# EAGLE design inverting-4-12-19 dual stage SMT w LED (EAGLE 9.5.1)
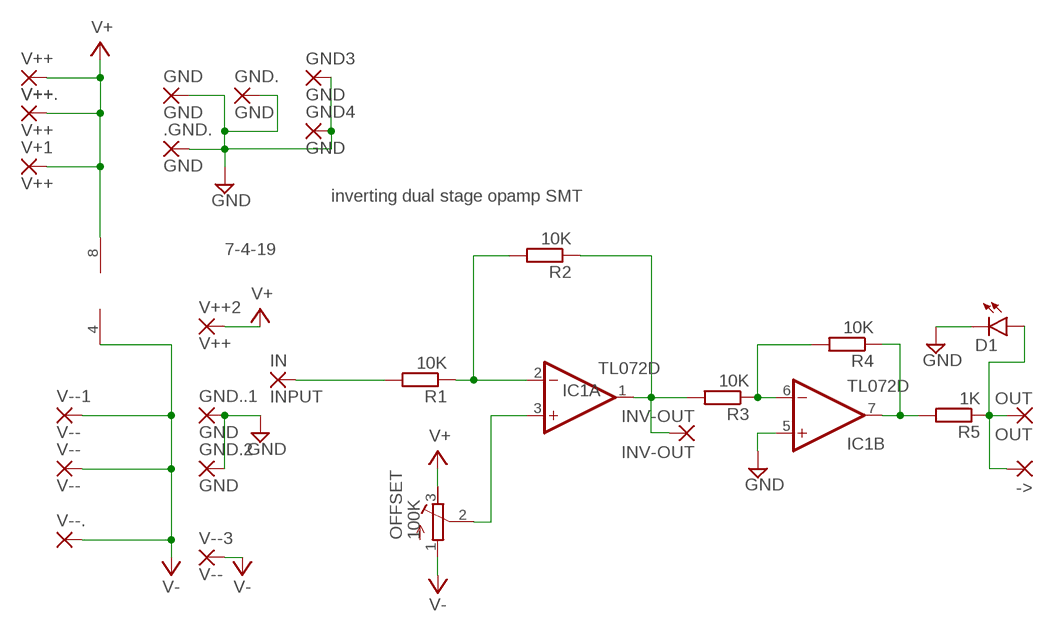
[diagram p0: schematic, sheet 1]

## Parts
->  1,6/0,8  [1,6/0,8]
.GND.  GND  1,6/0,9  [1,6/0,9]
D1  LED3MM  [LED3MM]
GND  GND  1,6/0,8  [1,6/0,8]
GND3  GND  1,6/0,8  [1,6/0,8]
GND4  GND  1,6/0,8  [1,6/0,8]
GND.  GND  1,6/0,8  [1,6/0,8]
GND.2  GND  1,6/0,8  [1,6/0,8]
GND..1  GND  1,6/0,8  [1,6/0,8]
IC1  TL072D  [SO08]
IN  INPUT  1,6/0,8  [1,6/0,8]
INV-OUT  INV-OUT  1,6/0,8  [1,6/0,8]
OFFSET  100K  R-TRIMM64W  [RTRIM64W]
OUT  OUT  1,6/0,8  [1,6/0,8]
R1  10K  RESISTORVERTICAL  [VERTICAL_RESISTOR]
R2  10K  RESISTORVERTICAL  [VERTICAL_RESISTOR]
R3  10K  RESISTORVERTICAL  [VERTICAL_RESISTOR]
R4  10K  RESISTORVERTICAL  [VERTICAL_RESISTOR]
R5  1K  RESISTORVERTICAL  [VERTICAL_RESISTOR]
V+1  V++  1,6/0,8  [1,6/0,8]
V++  V++  1,6/0,8  [1,6/0,8]
V++2  V++  1,6/0,8  [1,6/0,8]
V++.  V++  1,6/0,8  [1,6/0,8]
V--  V--  1,6/0,8  [1,6/0,8]
V--1  V--  1,6/0,8  [1,6/0,8]
V--3  V--  1,6/0,8  [1,6/0,8]
V--.  1,6/0,8  [1,6/0,8]

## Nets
GND: .GND..1(P) D1.K(C) GND3.1(P) GND4.1(P) GND.1(P) GND.2.1(P) GND..1(P) GND..1.1(P) IC1.5(B:+IN)
N$1: IC1.3(A:+IN) OFFSET.2(S)
N$2: ->.1(P) D1.A OUT.1(P) R5.1
N$3: IN.1(P) R1.2
N$5: IC1.2(A:-IN) R1.1 R2.2
N$6: IC1.6(B:-IN) R3.1 R4.2
N$7: IC1.7(B:OUT) R4.1 R5.2
N$18: IC1.1(A:OUT) INV-OUT.1(P) R2.1 R3.2
V+: IC1.8(P:V+) OFFSET.3(E) V+1.1(P) V++2.1(P) V++.1(P) V++..1(P)
V-: IC1.4(P:V-) OFFSET.1(A) V--1.1(P) V--3.1(P) V--.1(P) V--..1(P)

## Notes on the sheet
- inverting dual stage opamp SMT
- 7-4-19

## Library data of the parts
-> GND GND. IN INV-OUT OUT V++ V++. V-- V--. = wirepad:1,6/0,8: THROUGH-HOLE PAD
.GND. = wirepad:1,6/0,9: THROUGH-HOLE PAD
D1 = diodes:LED
GND3 GND4 GND.2 GND..1 V+1 V++2 V--1 V--3 = wirepad-NONAMES:1,6/0,8: THROUGH-HOLE PAD
IC1 = linear:TL072: OP AMP
OFFSET = rcl:R-TRIMM: Trimm resistor; SPICEMODEL: X; SPICEPREFIXL: POT
R1-R5 = MusicThingModular:RESISTOR: Standard resistor, various versions

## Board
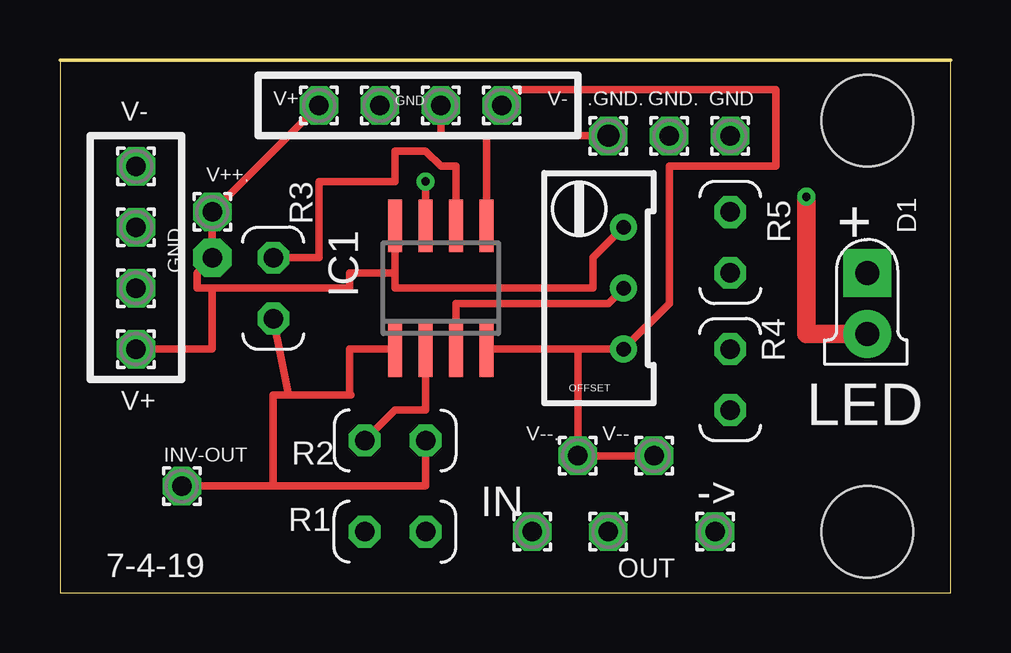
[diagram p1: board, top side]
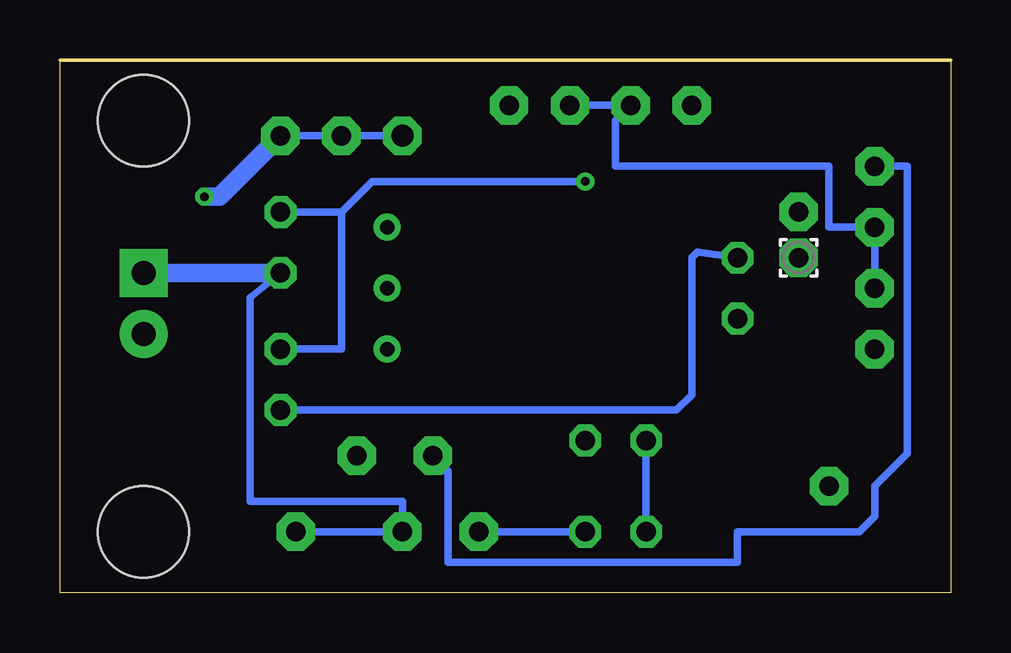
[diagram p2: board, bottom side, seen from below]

Size 37.14 x 22.21 mm. Coordinates in mm from the lower left corner, seen from the top.
Outline: 0,0 37.14,0 37.14,22.21 0,22.21 0,0
Copper layers (1*16): Top 0.035mm / dielectric 1.5mm / Bottom 0.035mm
Design rules "default": minimum track width 6mil, minimum drill 0.35mm, track to track 6mil, track to pad 6mil, pad to pad 6mil, via to via 6mil, smd to smd 6mil, copper to edge 40mil, drill to drill 6mil, minimum pad ring 10mil, minimum via ring 8mil, stop-mask expansion 4mil, vias tented up to drill 0mil, thermal gap 10mil
Holes 3.81 mm at 33.66,19.68 33.66,2.54

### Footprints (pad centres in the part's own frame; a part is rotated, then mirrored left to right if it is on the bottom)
1,6/0,8 = drill 0.813 pad 1.6 octagon: 1 0,0
1,6/0,9 = drill 0.914 pad 1.6 octagon: 1 0,0
LED3MM = drill 1 pad 2 square: A -1.27,0 | drill 1 pad 2: K 1.27,0
SO08 = smd 0.6 x 2.2: 1 -1.905,-2.6; 2 -0.635,-2.6; 3 0.635,-2.6; 4 1.905,-2.6; 5 1.905,2.6; 6 0.635,2.6; 7 -0.635,2.6; 8 -1.905,2.6
RTRIM64W = drill 0.61: 1 1.27,-2.54; 2 1.27,0; 3 1.27,2.54
VERTICAL_RESISTOR = drill 0.813 octagon: 1 -1.27,0; 2 1.27,0

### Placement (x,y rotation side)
->  27.3,2.54 0 top
.GND.  22.86,19.05 0 top
D1  33.66,12.06 270 top
GND  27.94,19.05 0 top
GND3  13.33,20.32 0 top
GND4  15.88,20.32 0 top
GND.  25.4,19.05 0 top
GND.2  3.17,12.7 0 top
GND..1  3.17,15.24 0 top
IC1  15.88,12.7 0 top
IN  19.68,2.54 0 top
INV-OUT  5.08,4.45 0 top
OFFSET  22.22,12.7 0 top
OUT  22.86,2.54 0 top
R1  13.97,2.54 0 top
R2  13.97,6.35 180 top
R3  8.89,12.7 270 top
R4  27.94,8.89 270 top
R5  27.94,14.6 90 top
V+1  10.79,20.32 0 top
V++  6.35,13.97 0 bottom
V++2  3.17,10.16 0 top
V++.  6.35,15.87 0 top
V--  24.76,5.71 0 top
V--1  18.41,20.32 0 top
V--3  3.17,17.78 0 top
V--.  21.59,5.71 0 top

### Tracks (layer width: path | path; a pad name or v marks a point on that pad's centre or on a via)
GND  (via drill 0.35)
  Top 0.305: IC1.5 17.78,19.05 | .GND..1 17.78,19.05 | 17.78,19.05 15.88,19.05 GND4.1
  Top 0.762: D1.K 31.11,10.79 v31.11,16.51
  Bottom 0.305: .GND..1 GND..1 GND.1 | GND4.1 GND3.1 13.97,19.68 13.97,17.78 5.08,17.78 5.08,15.24 GND..1.1 GND.2.1
  Bottom 0.762: GND.1 30.48,16.51 v31.11,16.51
N$1
  Top 0.305: IC1.3 16.51,12.06 22.86,12.06 OFFSET.2
N$2
  Bottom 0.305: R5.1 29.21,12.32 29.21,3.81 22.86,3.81 OUT.1 ->.1
  Bottom 0.762: R5.1 D1.A
N$3
  Bottom 0.305: R1.2 IN.1
N$5
  Top 0.305: R2.2 13.97,7.62 15.24,7.62 IC1.2
  Bottom 0.305: R1.1 R2.2
N$6
  Top 0.305: IC1.6 16.51,17.78 15.88,17.78 15.24,18.41 13.97,18.41 13.97,17.15 10.79,17.15 10.79,13.97 R3.1
  Bottom 0.305: R4.2 11.43,7.62 10.79,8.26 10.79,13.97 10.56,14.21 R3.1
N$7  (via drill 0.35)
  Top 0.305: IC1.7 v15.24,17.15
  Bottom 0.305: v15.24,17.15 24.13,17.15 25.4,15.87 | 25.4,15.87 25.4,10.16 R4.1 | R5.2 25.4,15.87
N$18
  Top 0.305: 9.52,8.26 R3.2 | INV-OUT.1 8.89,4.45 | 8.89,4.45 15.24,4.45 R2.1 | 8.89,4.45 8.89,8.26 9.52,8.26 | 9.52,8.26 12.12,8.26 12.06,8.31 12.06,10.16 13.91,10.16 IC1.1
V+
  Top 0.305: IC1.8 13.97,13.34 | 13.97,13.34 13.97,12.7 22.22,12.7 22.22,13.97 OFFSET.3 | 6.35,12.7 12.06,12.7 12.06,13.34 13.97,13.34 | 6.35,12.7 5.72,12.7 5.72,13.34 V++.1 V++..1 V+1.1 | V++2.1 6.35,10.16 6.35,12.7
V-
  Top 0.305: 21.59,10.16 V--..1 V--.1 | 21.59,10.16 OFFSET.1 25.4,12.06 25.4,17.78 29.85,17.78 29.85,20.97 19.06,20.97 V--1.1 | IC1.4 17.84,10.16 21.59,10.16
  Bottom 0.305: V--..1 21.59,5.08 20.95,5.08 20.95,1.27 8.89,1.27 8.89,2.54 3.81,2.54 3.17,3.17 3.17,4.45 1.8,5.82 1.8,17.78 V--3.1

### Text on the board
tNames: V- | V+ | GND | V- | + | GND | V+ | LED | 7-4-19
tValues: DUAL INVERTING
